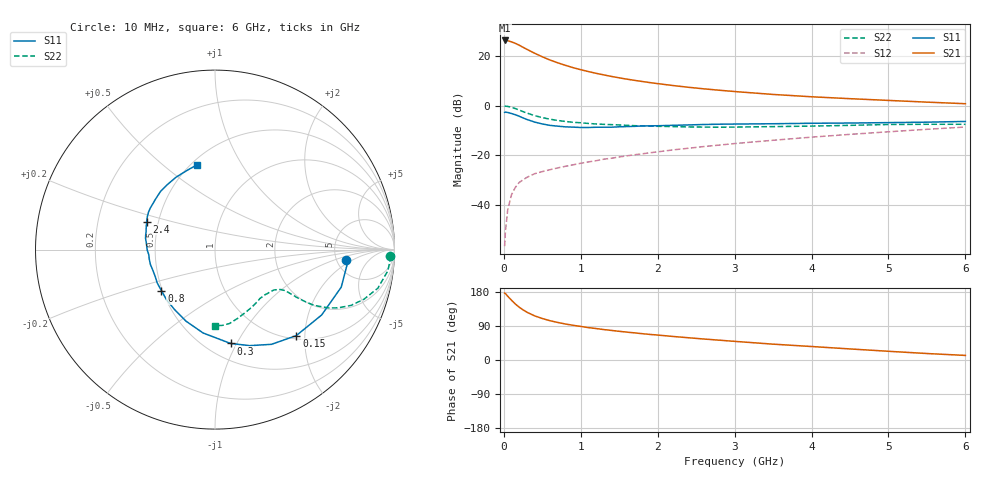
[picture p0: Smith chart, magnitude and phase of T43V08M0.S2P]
! Infineon Technologies  Discrete & RF Semiconductors
! BFR182T
! Si NPN RF Bipolar Junction Transistor in SC75
! VCE = 3 V  IC = 8 mA
! Common Emitter S-Parameters:  October  1999
# GHz  S  MA  R  50
!  f  S11  S21  S12  S22
! GHz  MAG  ANG  MAG  ANG  MAG  ANG  MAG  ANG
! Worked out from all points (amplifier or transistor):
!   36 points, 10 MHz to 6 GHz, reference 50 ohm
!   highest |S21| = 26.3 dB at 10 MHz (marker M1)
!   |S21| within 3 dB of that: start of sweep to 265.3 MHz
!   unconditionally stable (mu >= 1): 1.11 GHz to 3.858 GHz
!   at 250 MHz: K = 0.39, MSG = 26.6 dB, |S12| = -29.8 dB
!   at 1.4 GHz: K = 1.06, MAG = 14.9 dB, |S12| = -21.1 dB
!   at 6 GHz: K = 0.84, MSG = 4.7 dB, |S12| = -8.6 dB
!   lowest NFmin = 1.40 dB at 450 MHz
!   S11 on the Smith chart (normalised r, x): 10 MHz: 6.13, -1.53; 150 MHz: 1.07, -1.81; 300 MHz: 0.65, -0.94; 800 MHz: 0.49, -0.26; 2.4 GHz: 0.43, +0.16; 6 GHz: 0.54, +0.66
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0.01  0.734 -4.5  20.55 176.7  0.0015 78.2  0.9778 -2.1
0.02  0.7435 -5.2  20.54 175.5  0.0029 94.5  0.9801 -2.8
0.05  0.7337 -16.6  20.3 168.3  0.008 85.5  0.9701 -7.0
0.1  0.697 -31.5  19.25 157.7  0.0163 76.7  0.9328 -13.3
0.15  0.6594 -46.6  17.94 147.6  0.0229 69.2  0.8752 -18.4
0.2  0.6145 -59.2  16.49 139.3  0.0287 65.8  0.819 -22.3
0.25  0.5687 -70.2  14.98 132.3  0.0324 62.0  0.7616 -25.2
0.3  0.5299 -80.6  13.62 126.1  0.0363 60.8  0.7139 -27.1
0.4  0.4694 -98.1  11.38 116.5  0.043 56.9  0.6325 -29.4
0.5  0.4301 -112.1  9.646 109.5  0.0474 56.7  0.5777 -30.0
0.6  0.4028 -124.1  8.308 103.7  0.0517 56.2  0.5364 -30.3
0.7  0.3885 -134.0  7.306 99.1  0.0562 57.7  0.5058 -30.3
0.8  0.3764 -142.4  6.504 95.0  0.0605 57.8  0.4833 -30.3
1.1  0.3654 -162.6  4.863 85.4  0.0742 60.3  0.4408 -30.8
1.4  0.3702 -175.8  3.882 78.0  0.088 62.2  0.4169 -32.5
1.6  0.3815 176.5  3.424 73.5  0.0983 63.1  0.4032 -33.7
2.2  0.4037 161.6  2.549 62.1  0.1294 64.7  0.3812 -39.9
2.4  0.4114 157.8  2.351 58.7  0.1398 65.0  0.3748 -42.4
3.5  0.4347 139.6  1.688 41.8  0.2022 63.0  0.3803 -57.0
4.5  0.4491 126.2  1.387 29.2  0.2657 59.2  0.4033 -71.8
5.5  0.4675 109.7  1.182 17.1  0.3359 53.8  0.4243 -84.7
6  0.4836 101.7  1.099 12.1  0.3731 50.3  0.4237 -90.1
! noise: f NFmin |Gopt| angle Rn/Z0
0.45  1.4  0.26  41  0.29
0.9  1.5  0.25  83  0.23
1.8  2  0.21  162  0.2
